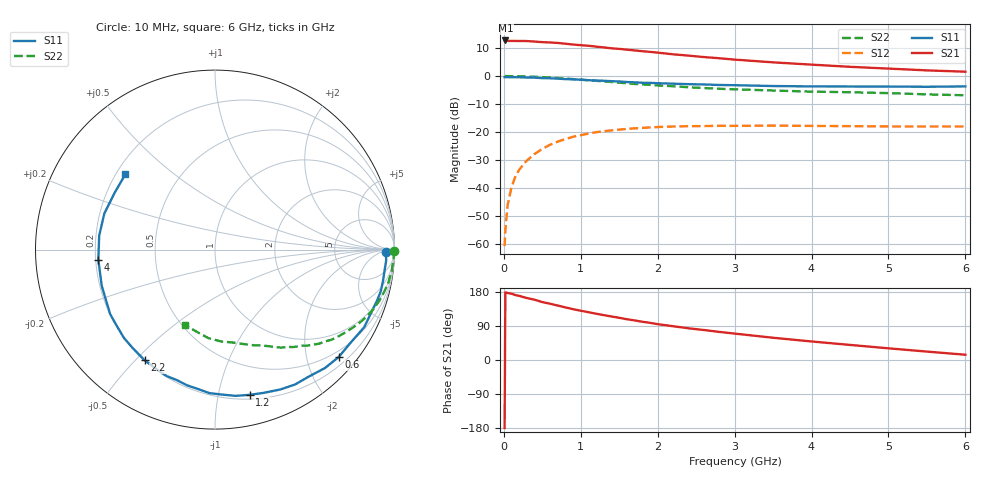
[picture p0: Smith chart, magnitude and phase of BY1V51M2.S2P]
! SIEMENS Small Signal Semiconductors
! BFY420
! Si NPN RF SIEGET Grounded Emitter Transistor in MICRO-X
! VCE = 1.5 V  IC = 1.2 mA
! Common Emitter S-Parameters:  October  1996
# GHz  S  MA  R  50
!  f  S11  S21  S12  S22
! GHz  MAG  ANG  MAG  ANG  MAG  ANG  MAG  ANG
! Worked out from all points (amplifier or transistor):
!   36 points, 10 MHz to 6 GHz, reference 50 ohm
!   highest |S21| = 12.7 dB at 20 MHz (marker M1)
!   |S21| within 3 dB of that: start of sweep to 1.491 GHz
!   unconditionally stable (mu >= 1): 4.448 GHz to end of sweep
!   at 250 MHz: K = 0.04, MSG = 22.2 dB, |S12| = -31.8 dB
!   at 1.4 GHz: K = 0.23, MSG = 14.7 dB, |S12| = -19.5 dB
!   at 6 GHz: K = 1.32, MAG = 6.4 dB, |S12| = -18.0 dB
!   S11 on the Smith chart (normalised r, x): 10 MHz: 39, -11; 600 MHz: 0.37, -2.63; 1.2 GHz: 0.24, -1.24; 2.2 GHz: 0.20, -0.53; 4 GHz: 0.21, -0.04; 6 GHz: 0.24, +0.35
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0.01  0.9537 -0.8  4.33 -179.4  0.0009 110.8  0.9995 -0.3
0.02  0.9519 -1.6  4.337 178.7  0.0018 88.3  0.9976 -0.7
0.05  0.9559 -3.5  4.257 176.8  0.005 86.7  0.9972 -1.8
0.1  0.9519 -7.1  4.254 175.0  0.0103 85.4  0.9958 -3.6
0.15  0.9522 -10.4  4.249 171.2  0.0159 83.2  0.9926 -5.4
0.2  0.9525 -14.0  4.234 169.3  0.021 82.7  0.9918 -7.1
0.3  0.9401 -20.7  4.226 163.5  0.0308 77.2  0.9835 -10.7
0.4  0.9371 -27.5  4.145 159.1  0.0403 73.5  0.971 -14.2
0.5  0.9167 -34.3  4.044 152.8  0.0497 69.3  0.9577 -17.5
0.6  0.9129 -41.0  3.995 148.5  0.0588 65.1  0.9409 -20.9
0.8  0.88 -53.3  3.791 138.8  0.0745 57.6  0.9019 -27.0
1.1  0.8428 -71.3  3.487 126.1  0.0932 47.8  0.8408 -35.1
1.2  0.8319 -76.6  3.361 122.1  0.0988 44.6  0.8209 -37.7
1.5  0.8003 -92.2  3.064 111.4  0.11 36.2  0.7612 -44.1
1.8  0.7577 -106.2  2.783 100.9  0.118 29.4  0.7092 -49.5
2.2  0.7303 -122.5  2.45 89.1  0.1249 21.7  0.6571 -56.2
2.8  0.6922 -142.6  2.084 74.2  0.1285 13.5  0.5919 -64.5
3.5  0.6624 -162.4  1.759 58.7  0.1297 6.7  0.55 -73.1
4  0.6525 -175.1  1.601 48.9  0.128 3.4  0.5262 -79.5
4.5  0.6499 173.1  1.463 39.8  0.1268 0.4  0.513 -86.2
5.5  0.6426 150.3  1.263 22.2  0.1251 -1.9  0.4698 -102.2
6  0.6524 139.9  1.196 13.9  0.1252 -2.0  0.4526 -111.3
